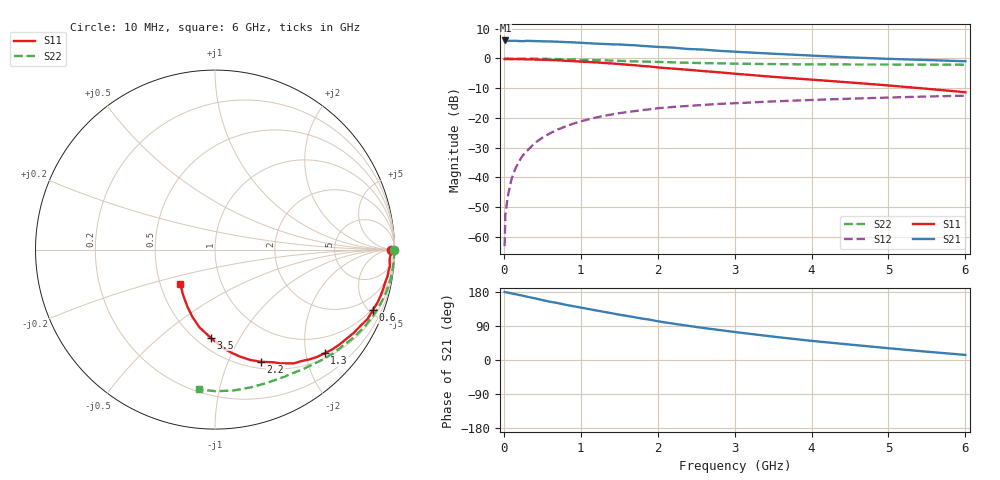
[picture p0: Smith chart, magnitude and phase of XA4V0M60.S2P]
! SIEMENS Discrete & RF Semiconductors
! BFY180
! Si NPN RF Bipolar Junction Transistor in MICRO-X
! VCE = 4 V  IC = 0.6 mA
! Common Emitter S-Parameters:  May  1997
# GHz  S  MA  R  50
!  f  S11  S21  S12  S22
! GHz  MAG  ANG  MAG  ANG  MAG  ANG  MAG  ANG
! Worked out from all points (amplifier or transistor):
!   36 points, 10 MHz to 6 GHz, reference 50 ohm
!   highest |S21| = 6.1 dB at 20 MHz (marker M1)
!   |S21| within 3 dB of that: start of sweep to 2.521 GHz
!   unconditionally stable (mu >= 1): 5.244 GHz to end of sweep
!   at 250 MHz: K = 0.07, MSG = 19.1 dB, |S12| = -32.5 dB
!   at 1.4 GHz: K = 0.41, MSG = 11.8 dB, |S12| = -18.8 dB
!   at 6 GHz: K = 1.02, MAG = 4.8 dB, |S12| = -12.5 dB
!   S11 on the Smith chart (normalised r, x): 10 MHz: 94, -16; 600 MHz: 0.87, -5.28; 1.3 GHz: 0.60, -2.38; 2.2 GHz: 0.58, -1.32; 3.5 GHz: 0.59, -0.76; 6 GHz: 0.63, -0.26
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0.01  0.9795 -0.2  1.971 179.6  0.0007 93.6  0.9991 -0.1
0.02  0.9702 -0.8  2.009 178.9  0.0024 92.5  0.9999 -0.6
0.05  0.9783 -1.6  1.983 178.0  0.0047 86.8  0.9985 -1.2
0.1  0.9745 -3.5  1.976 175.9  0.0094 89.3  0.998 -2.4
0.2  0.9744 -6.9  1.963 171.5  0.0189 84.6  0.9963 -4.7
0.25  0.9725 -8.8  1.953 169.6  0.0238 83.3  0.9974 -5.9
0.3  0.967 -10.5  1.981 167.1  0.0279 81.7  0.9939 -7.0
0.4  0.9608 -14.0  1.962 162.9  0.0377 79.5  0.9925 -9.3
0.6  0.9428 -20.9  1.933 153.7  0.0552 74.2  0.9828 -13.9
0.8  0.9152 -27.7  1.887 145.8  0.0719 69.2  0.969 -18.4
1.1  0.873 -37.1  1.805 134.6  0.0947 61.7  0.9467 -24.6
1.3  0.8409 -43.4  1.756 127.2  0.1087 57.1  0.9302 -28.8
1.5  0.8085 -49.1  1.72 119.6  0.1203 52.9  0.9131 -32.6
1.7  0.7711 -55.3  1.667 112.9  0.1302 49.1  0.8924 -36.3
2.2  0.6753 -67.7  1.521 96.0  0.1532 40.6  0.8621 -44.7
2.6  0.6124 -76.8  1.409 84.3  0.166 35.3  0.8363 -50.6
3  0.5551 -84.6  1.3 73.9  0.1767 30.2  0.8186 -56.1
3.5  0.4913 -92.9  1.202 61.7  0.1899 25.2  0.8047 -62.6
4  0.4411 -101.4  1.119 50.5  0.2008 20.2  0.7965 -69.2
4.5  0.3954 -108.6  1.044 40.7  0.2111 15.8  0.7929 -75.9
5.5  0.3093 -125.1  0.942 21.9  0.2295 7.1  0.789 -89.7
6  0.2713 -135.3  0.898 13.5  0.2373 2.5  0.7841 -96.6
